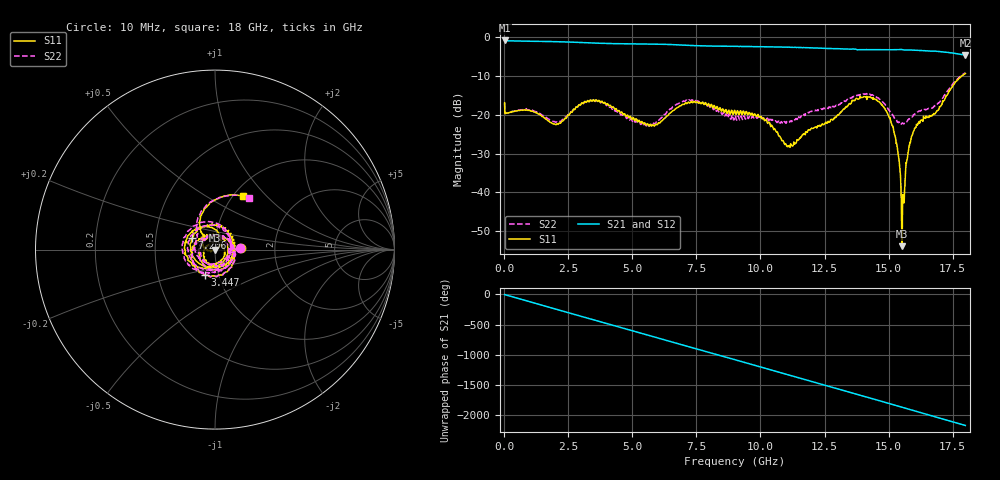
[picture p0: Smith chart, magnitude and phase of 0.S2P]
!Agilent Technologies,E5071C,MY46316741,A.11.02
!Date: Tue Sep 22 10:02:19 2020
!Data & Calibration Information:
!Freq	S11:SOLT4(ON)	S21:SOLT4(ON)	S12:SOLT4(ON)	S22:SOLT4(ON)
!PortZ  Port1:50+j0  Port2:50+j0
!Above PortZ is port z conversion or system Z0 setting when saving the data.
!When reading, reference impedance value at option line is always used.
# Hz S dB R 50
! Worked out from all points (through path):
!   1561 points, 10 MHz to 18 GHz, reference 50 ohm
!   highest |S21| = -0.92 dB at 10 MHz (marker M1); lowest = -4.7 dB at 18 GHz (marker M2)
!   group delay of S21, straight-line fit = 336 ps
!   lowest |S11| = -53.8 dB at 15.53 GHz (marker M3), VSWR 1.00, Z = 50 - j0.201 ohm
!   |S11| at or under -10 dB: start of sweep to 17.87 GHz
!   |S22| runs from -23.0 to -9.2 dB; largest |S21 - S12| = 0.015
!   S11 on the Smith chart (normalised r, x): 10 MHz: 1.33, +0.02; 3.447 GHz: 0.86, -0.25; 7.206 GHz: 0.77, +0.10; 18 GHz: 1.10, +0.75
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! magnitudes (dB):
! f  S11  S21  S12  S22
! 10 MHz  -16.9  -0.9  -0.9  -17.1
! 2.04 GHz  -22.4  -1.2  -1.2  -21.8
! 3.02 GHz  -17.0  -1.5  -1.5  -17.1
! 3.447 GHz  -16.3  -1.6  -1.6  -16.5
! 5.384 GHz  -21.9  -1.8  -1.8  -22.2
! 6.007 GHz  -22.2  -1.9  -1.9  -21.6
! 7.206 GHz  -16.8  -2.2  -2.2  -16.2
! 9.005 GHz  -19.1  -2.4  -2.5  -20.3
! 10.05 GHz  -21.0  -2.5  -2.5  -20.8
! 11.08 GHz  -28.1  -2.6  -2.6  -21.7
! 12.01 GHz  -23.5  -2.8  -2.8  -19.0
! 13.98 GHz  -15.6  -3.3  -3.3  -14.8
! 14.57 GHz  -16.5  -3.3  -3.3  -15.7
! 15 GHz  -20.3  -3.3  -3.3  -18.7
! 15.34 GHz  -28.2  -3.3  -3.3  -21.8
! 15.53 GHz  -53.8  -3.3  -3.3  -22.2
! 15.59 GHz  -41.6  -3.4  -3.3  -22.4
! 15.64 GHz  -38.4  -3.4  -3.3  -22.0
! 15.76 GHz  -29.8  -3.4  -3.3  -21.3
! 16.03 GHz  -23.5  -3.4  -3.5  -19.8
! 16.9 GHz  -18.9  -3.7  -3.8  -17.3
! 18 GHz  -9.4  -4.7  -4.7  -9.2
